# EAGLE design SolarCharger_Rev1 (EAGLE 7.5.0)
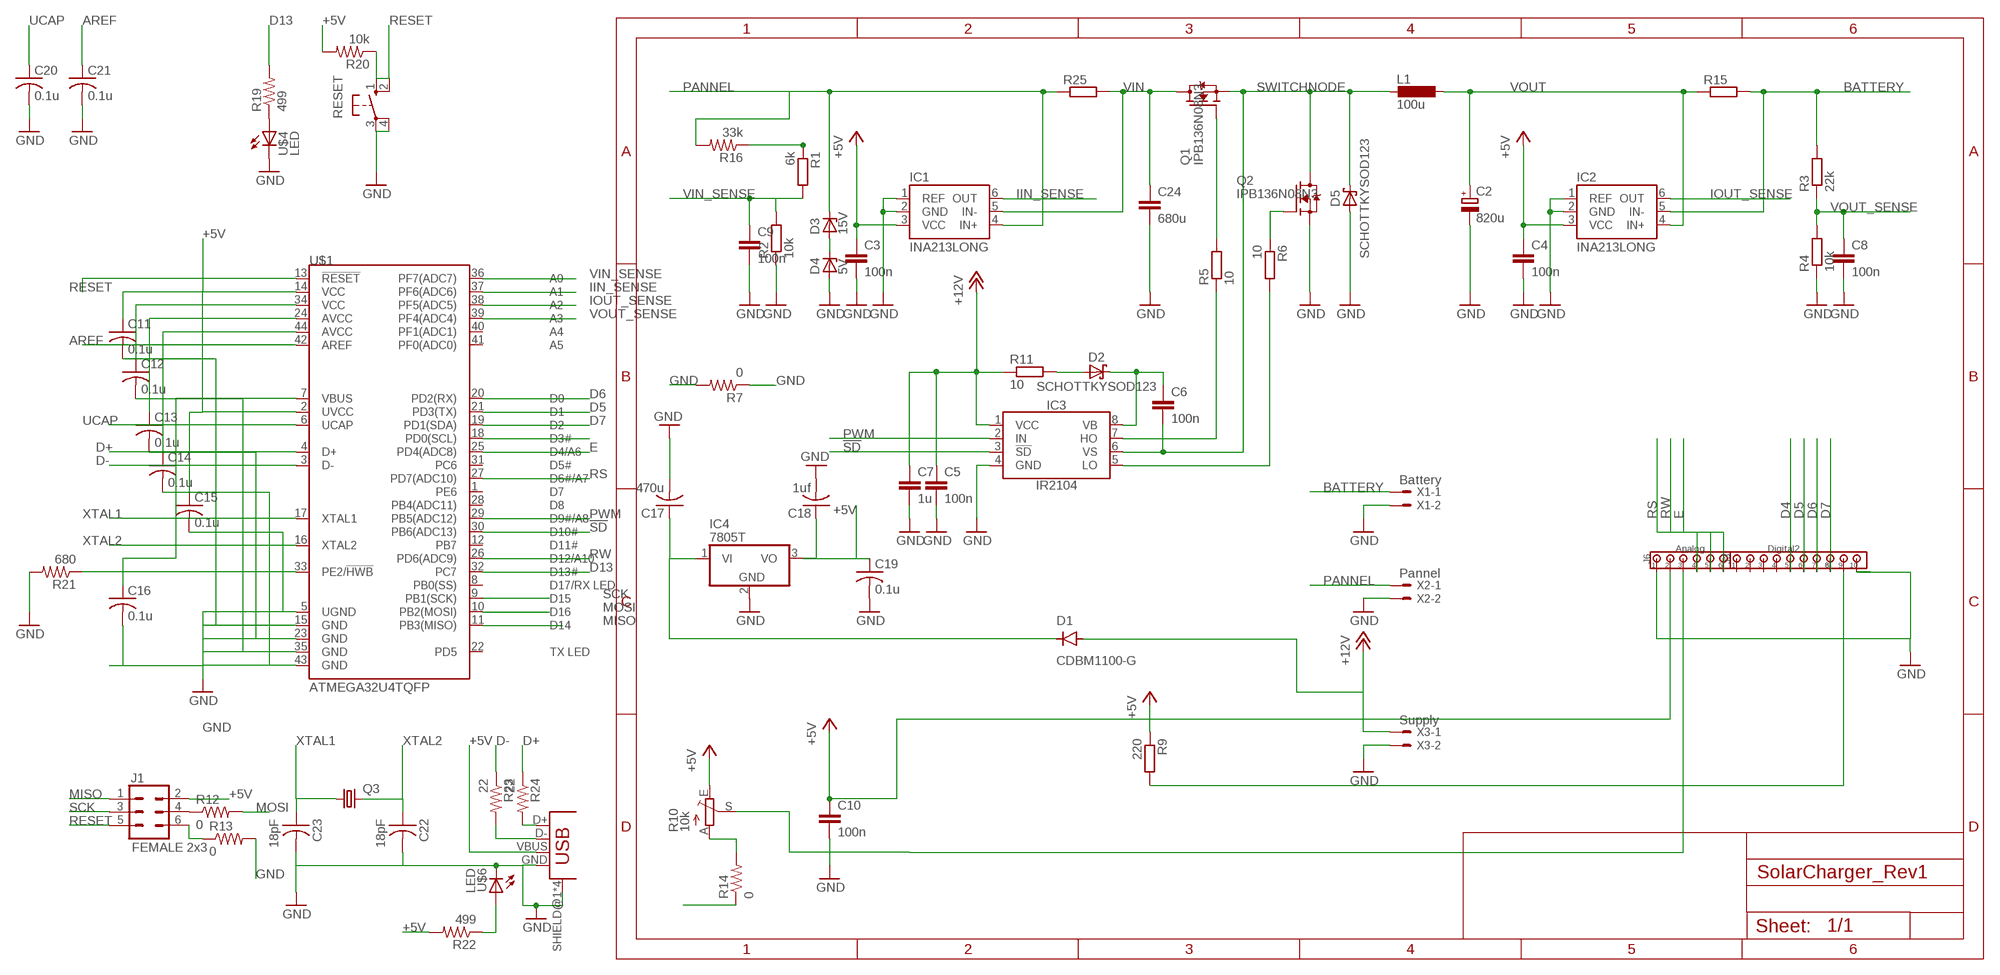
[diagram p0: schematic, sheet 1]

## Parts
C2  820u  C_POLARIZED10MM  [10MM]
C3  100n  CC0805  [C0805]
C4  100n  CC0805  [C0805]
C5  100n  CC0805  [C0805]
C6  100n  CC0805  [C0805]
C7  1u  CC0805  [C0805]
C8  100n  CC0805  [C0805]
C9  100n  CC0805  [C0805]
C10  100n  CC0805  [C0805]
C11  0.1u  C-USC1206  [C1206]
C12  0.1u  C-USC1206  [C1206]
C13  0.1u  C-USC1206  [C1206]
C14  0.1u  C-USC1206  [C1206]
C15  0.1u  C-USC1206  [C1206]
C16  0.1u  C-USC1206  [C1206]
C17  470u  C-USC1206  [C1206]
C18  1uf  C-USC1206  [C1206]
C19  0.1u  C-USC1206  [C1206]
C20  0.1u  C-USC1206  [C1206]
C21  0.1u  C-USC1206  [C1206]
C22  18pF  CAP-US1206FAB  [C1206FAB]
C23  18pF  CAP-US1206FAB  [C1206FAB]
C24  680u  10NF-PTH-10MM-10000V-1-%  [CAP-PTH-10MM]
D1  CDBM1100-G  [MINI-SMA]
D2  SCHOTTKYSOD123  [SOD123]
D3  15V  ZENER-DIODEDO41Z10  [DO41Z10]
D4  5V  ZENER-DIODEDO41Z10  [DO41Z10]
D5  SCHOTTKYSOD123  [SOD123]
IC1  INA213LONG  [SC70-6_LONG]
IC2  INA213LONG  [SC70-6_LONG]
IC3  IR2104  [SOIC8]
IC4  7805T  [TO220H]
J1  FEMALE 2x3  CONN_03X2FEMALE  [2X3]
J3  Digital2  100MIL_10X  [100MIL_10X_ROUND]
J6  Analog  100MIL_6X  [100MIL_6X_ROUND]
L1  100u  L-EU0207/12  [0207/12]
Q1  IPB136N08N3  N-PWR-MOSFETTO263-3  [TO263-3]
Q2  IPB136N08N3  IPB136N08N3_GTO263  [TO263-3@1]
Q3  CRYSTALTC26V  [TC26V]
R1  6k  R-EU_M1206  [M1206]
R2  10k  R-EU_M1206  [M1206]
R3  22k  R-EU_M1206  [M1206]
R4  10k  R-EU_M1206  [M1206]
R5  10  R-EU_M1206  [M1206]
R6  10  R-EU_M1206  [M1206]
R7  0  RES-US1206FAB  [R1206FAB]
R9  220  R-EU_M1206  [M1206]
R10  10k  TRIM_EU-B25X  [B25X]
R11  10  R-EU_M1206  [M1206]
R12  0  RES-US1206FAB  [R1206FAB]
R13  0  RES-US1206FAB  [R1206FAB]
R14  0  RES-US1206FAB  [R1206FAB]
R15  SMR  [SMR]
R16  33k  RES-US1206FAB  [R1206FAB]
R19  499  RES-US1206  [R1206]
R20  10k  RES-US1206  [R1206]
R21  680  RES-US1206  [R1206]
R22  499  RES-US1206  [R1206]
R23  22  RES-US1206  [R1206]
R24  22  RES-US1206  [R1206]
R25  SMR  [SMR]
RESET  10-XX  [B3F-10XX]
U$1  ATMEGA32U4TQFP  [SPARKFUN-DIGITALIC_TQFP44]
U$4  LED  [LED1206]
U$5  USB_MINIB  [USB_MINIB]
U$6  LED  [LED1206]
X1  Battery  22-23-2021200MIL  [200MIL_2X]
X2  Pannel  22-23-2021200MIL  [200MIL_2X]
X3  Supply  22-23-2021100MIL  [22-23-2021]

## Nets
!SD!: IC3.3(!SD!) U$1.30(PB6(ADC13))
+5V: C3.1 C4.1 C10.1 C11.1 C12.1 C13.1 C14.1 C15.1 C16.1 C18.1 C19.1 IC1.3(VCC) IC2.3(VCC) IC4.3(VO) J1.2 J6.2 R9.1 R10.E R20.2 R22.2 U$1.2(UVCC) U$1.7(VBUS) U$1.14(VCC) U$1.24(AVCC) U$1.34(VCC) U$1.44(AVCC) U$5.VBUS
+12V: C5.1 C7.1 D1.ANODE IC3.1(VCC) R11.1 X3.1
AREF: C21.1 U$1.42(AREF)
BATTERY: IC2.5(IN-) R3.2 R15.1 X1.1
D4: J3.5 U$1.18(PD0(SCL))
D5: J3.6 U$1.21(PD3(TX))
D6: J3.7 U$1.20(PD2(RX))
D7: J3.8 U$1.19(PD1(SDA))
D13: R19.2 U$1.32(PC7)
D+: R24.1 U$1.4(D+)
D-: R23.1 U$1.3(D-)
E: J6.6 U$1.25(PD4(ADC8))
GND: C2.- C3.2 C4.2 C5.2 C7.2 C8.2 C9.2 C10.2 C11.2 C12.2 C13.2 C14.2 C15.2 C16.2 C17.2 C18.2 C19.2 C20.2 C21.2 C22.2 C23.2 C24.2 D4.A D5.A IC1.1(REF) IC1.2(GND) IC2.1(REF) IC2.2(GND) IC3.4(GND) IC4.2(GND) J3.10 J6.1 Q2.3(S) R2.1 R4.1 R7.1 R7.2 R10.A R13.2 R14.1 R14.2 R21.2 RESET.3(P) RESET.4(P1) U$1.5(UGND) U$1.15(GND) U$1.23(GND) U$1.35(GND) U$1.43(GND) U$4.2(C) U$5.GND U$5.SHIELD@1(SHIELD) U$5.SHIELD@2(SHIELD) U$5.SHIELD@3(SHIELD) U$5.SHIELD@4(SHIELD) U$6.2(C) X1.2 X2.2 X3.2
IIN_SENSE: IC1.6(OUT) U$1.37(PF6(ADC6))
IOUT_SENSE: IC2.6(OUT) U$1.38(PF5(ADC5))
MISO: J1.1 U$1.11(PB3(MISO))
MOSI: R12.2 U$1.10(PB2(MOSI))
N$1: J1.4 R12.1
N$2: J1.6 R13.1
N$4: Q1.1(G) R5.2
N$7: Q2.1(G) R6.1
N$9: J3.9 R9.2
N$10: J6.3 R10.S
N$11: D2.A R11.2
N$12: C6.1 D2.C IC3.8(VB)
N$14: IC3.7(HO) R5.1
N$15: IC3.5(LO) R6.2
N$17: R1.1 R16.1
N$19: D3.A D4.C
N$20: C17.1 D1.KATHODE IC4.1(VI)
N$23: R19.1 U$4.1(A)
N$24: R21.1 U$1.33(PE2/!HWB)
N$25: R24.2 U$5.D+
N$26: R22.1 U$6.1(A)
N$27: R23.2 U$5.D-
PANNEL: D3.C IC1.4(IN+) R16.2 R25.2 X2.1
PWM: IC3.2(IN) U$1.29(PB5(ADC12))
RESET: J1.5 R20.1 RESET.1(S) RESET.2(S1) U$1.13(!RESET)
RS: J6.4 U$1.27(PD7(ADC10))
RW: J6.5 U$1.26(PD6(ADC9))
SCK: J1.3 U$1.9(PB1(SCK))
SWITCHNODE: C6.2 D5.C IC3.6(VS) L1.2 Q1.3(S) Q2.TAB(D)
UCAP: C20.1 U$1.6(UCAP)
VIN: C24.1 IC1.5(IN-) Q1.TAB(D) R25.1
VIN_SENSE: C9.1 R1.2 R2.2 U$1.36(PF7(ADC7))
VOUT: C2.+ IC2.4(IN+) L1.1 R15.2
VOUT_SENSE: C8.1 R3.1 R4.2 U$1.39(PF4(ADC4))
XTAL1: C23.1 Q3.1 U$1.17(XTAL1)
XTAL2: C22.1 Q3.2 U$1.16(XTAL2)
Unconnected: J3.1 J3.2 J3.3 J3.4 U$1.1(PE6) U$1.8(PB0(SS)) U$1.12(PB7) U$1.22(PD5) U$1.28(PB4(ADC11)) U$1.31(PC6) U$1.40(PF1(ADC1)) U$1.41(PF0(ADC0))

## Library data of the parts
C2 = 00Capacitor:C_POLARIZED
C3-C10 = 00Capacitor:C: Capacitor
C11-C21 = rcl:C-US: CAPACITOR, American symbol
C22 C23 = fab:CAP-US
C24 = SparkFun-Capacitors:10NF: 0.01uF/10nF/10,000pF ceramic capacitors; PROD_ID: CAP-09321; VALUE: 10nF
D1 = fab:CDBM1100-G: Diode schottky 100V 1A mini-SMA as found in the fablab inventory
D2 D5 = 00Diode:SCHOTTKY
D3 D4 = diode:ZENER-DIODE: Z-Diode
IC1 IC2 = 00Sensor:INA21*: Current-Shunt Monitors Voltage Output, Low- or High-Side Measurement, Bidirectional, Zero-Drift Series; GAIN: 50
IC3 = 00Logic:IR2104: Half-Bridge Driver Up to +600V Gate drive supply 10-20V Deadtime 520ns
IC4 = linear:78*: Positive VOLTAGE REGULATOR Source: http://cache.national.com/ds/LM/LM78L05.pdf http://www.fairchildsemi.com/ds/LM/LM7805.pdf
J1 = SparkFun-Connectors:CONN_03X2: Multi connection point. Often used as Generic Header-pin footprint for 0.1 inch spaced/style header connections You can populate with any combo of single row headers, but if you'd like an exact match, check these: Header - 2x3 (Male, 0.1") (PRT-12807) Header - 2x3 (Female, 0.1") (PRT-13010) 2x3 Pin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; PROD_ID: CONN-11566
J3 = 00Connector:100MIL_10X: 100mil 10-pin connector
J6 = 00Connector:100MIL_6X: 100 mil 6-pin connector
L1 = rcl:L-EU: INDUCTOR, European symbol
Q1 = 00Mosfet:N-PWR-MOSFET
Q2 = 00Mosfet:IPB136N08N3_G
Q3 = adafruit:CRYSTAL: CRYSTAL; OC_FARNELL: unknown; OC_NEWARK: unknown
R1-R6 R9 R11 = rcl:R-EU_: RESISTOR, European symbol
R7 R12-R14 R16 R19-R24 = fab:RES-US: Resistor (US Symbol)
R10 = pot:TRIM_EU-: POTENTIOMETER
R15 R25 = resistor-shunt:SMR: SMD SHUNT RESISTOR; OC_FARNELL: unknown; OC_NEWARK: unknown
RESET = switch-omron:10-XX: OMRON SWITCH; MPN: B3F-1000; OC_FARNELL: 176432; OC_NEWARK: 36M3542
U$1 = SparkFun-Retired:ATMEGA32U4: Atmel 44-pin 8-bit Microcontroller with 32KBytes of ISP Flash and USB Controller ----- Please use the QFN-44-NOPAD_1:1 package for the footprint of all boards using a 32U4. Route traces directly away from the pads as much as possible.; PROD_ID: IC-11161
U$4 U$6 = fab:LED: LED
U$5 = fab:USB_MINIB
X1 X2 = 00Connector:22-23-2021: .100" (2.54mm) Center Header - 2 Pin
X3 = 00Connector:22-23-2021: .100" (2.54mm) Center Header - 2 Pin; MF: MOLEX; MPN: 22-23-2021; OC_FARNELL: 1462926; OC_NEWARK: 25C3832

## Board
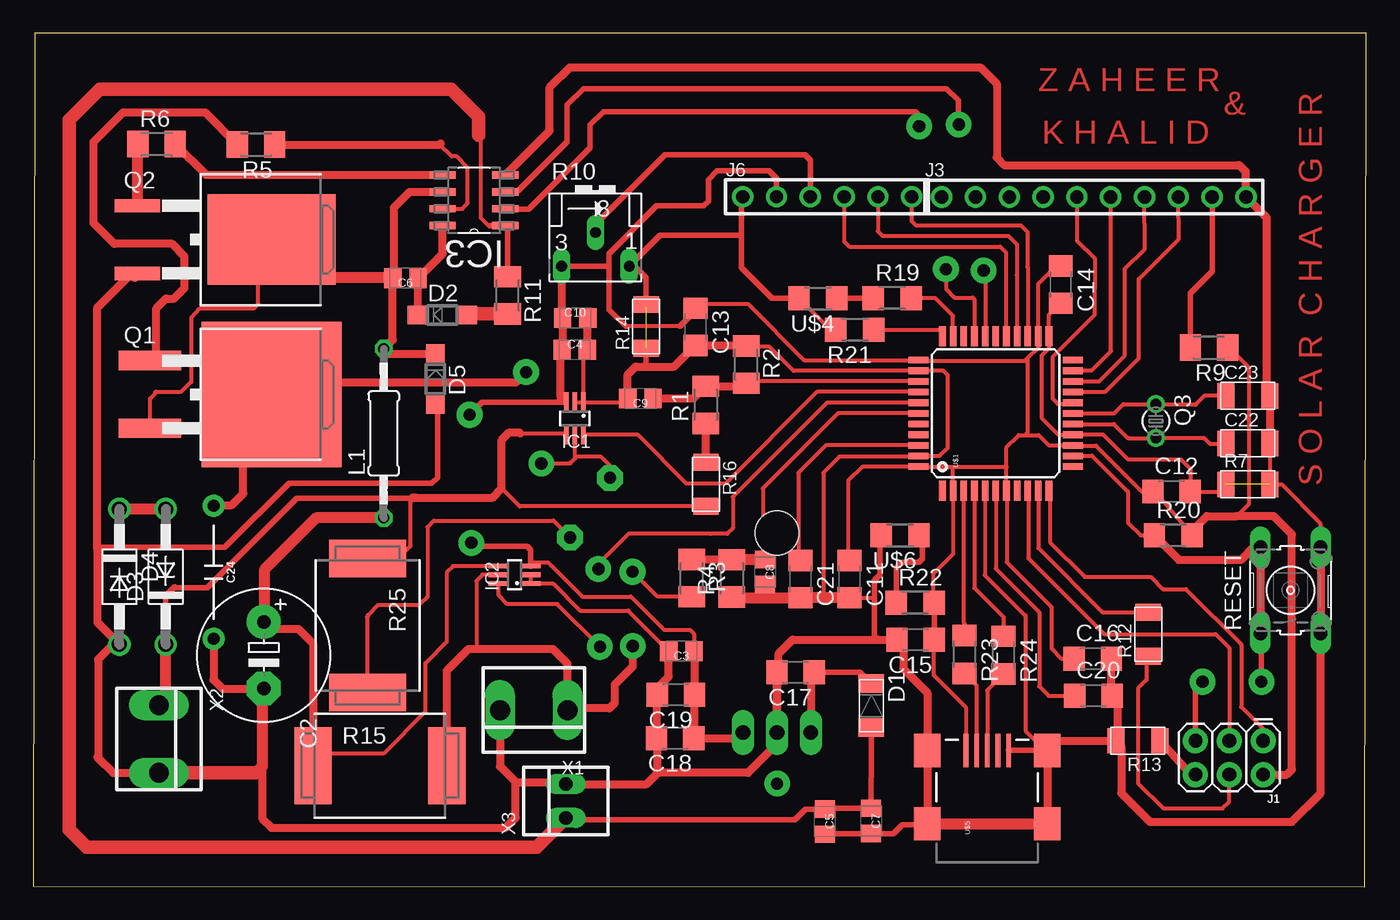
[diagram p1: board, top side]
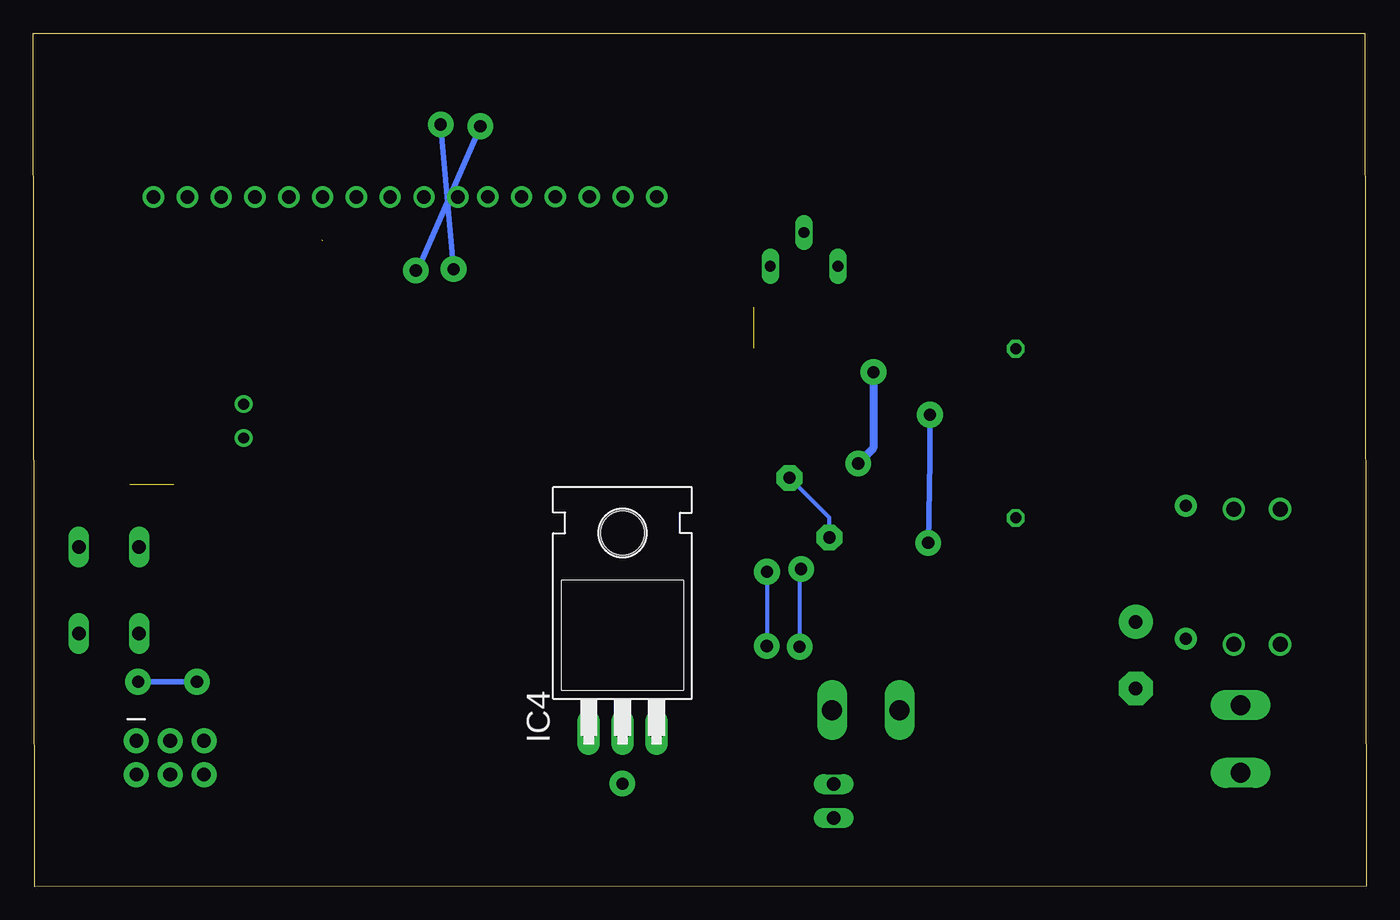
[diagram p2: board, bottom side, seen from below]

Size 100.15 x 64.08 mm. Coordinates in mm from the lower left corner, seen from the top.
Outline: 0,0.01 100.03,0 100.14,64.07 0.12,64.08 0,0.01
Copper layers (1*16): Top 0.035mm / dielectric 1.5mm / Bottom 0.035mm
Design rules "default": minimum track width 10mil, minimum drill 24mil, track to track 8mil, track to pad 8mil, pad to pad 8mil, via to via 8mil, smd to smd 8mil, copper to edge 40mil, drill to drill 8mil, minimum pad ring 10mil, minimum via ring 8mil, stop-mask expansion 4mil, vias tented up to drill 0mil, thermal gap 10mil

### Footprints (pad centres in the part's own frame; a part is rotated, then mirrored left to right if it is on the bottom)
10MM = drill 1.016 pad 2.54: + -2.5,0 | drill 1.016 pad 2.54 octagon: - 2.5,0
C0805 = smd 1.3 x 1.5: 1 -0.95,0; 2 0.95,0
C1206 = smd 1.6 x 1.8: 1 -1.4,0; 2 1.4,0
C1206FAB = smd 1.27 x 1.905: 1 -1.651,0; 2 1.651,0
CAP-PTH-10MM = drill 0.9 pad 1.651: 1 -5,0; 2 5,0
MINI-SMA = smd 1.4 x 1.9: ANODE 1.65,0; KATHODE -1.65,0
SOD123 = smd 1.4 x 1.4: A 1.9,0; C -1.9,0
DO41Z10 = drill 1.118: A 5.08,0; C -5.08,0
SC70-6_LONG = smd 0.35 x 1.5: 1 -0.65,-1.2; 2 0,-1.2; 3 0.65,-1.2; 4 0.65,1.2; 5 0,1.2; 6 -0.65,1.2
SOIC8 = smd 1.981 x 0.559: 1 -2.362,1.905; 2 -2.362,0.635; 3 -2.362,-0.635; 4 -2.362,-1.905; 5 2.362,-1.905; 6 2.362,-0.635; 7 2.362,0.635; 8 2.362,1.905
TO220H = drill 1.118 long: 1 -2.54,-10.16; 2 0,-10.16; 3 2.54,-10.16 | hole 3.302: 0,4.826
2X3 = drill 1.016 pad 1.88: 1 0,0; 2 0,2.54; 3 2.54,0; 4 2.54,2.54; 5 5.08,0; 6 5.08,2.54
100MIL_10X_ROUND = drill 1 pad 1.6: 1 -8.89,0; 2 -6.35,0; 3 -3.81,0; 4 -1.27,0; 5 1.27,0; 6 3.81,0; 7 6.35,0; 8 8.89,0; 9 11.43,0; 10 13.97,0
100MIL_6X_ROUND = drill 1 pad 1.6: 1 -6.35,0; 2 -3.81,0; 3 -1.27,0; 4 1.27,0; 5 3.81,0; 6 6.35,0
0207/12 = drill 0.813 octagon: 1 -6.35,0; 2 6.35,0
TO263-3 = smd 1.45 x 4.7: 1 -2.54,-5.65; 3 2.54,-5.65 | smd 10.9 x 10.5: TAB 0,3.5
TO263-3@1 = smd 1 x 3.4: 1 -2.54,-6.6; 3 2.54,-6.6 | smd 6.8 x 9.6: TAB 0,3.5
TC26V = drill 0.813: 1 -1.27,0; 2 1.27,0
M1206 = smd 1.6 x 2: 1 -1.4,0; 2 1.4,0
R1206FAB = smd 1.27 x 1.905: 1 -1.651,0; 2 1.651,0
B25X = drill 0.813 long: A 2.54,-1.905; E -2.54,-1.905; S 0,0.635
SMR = smd 2.8 x 5.8: 1 5.029,0; 2 -5.029,0
R1206 = smd 1.6 x 1.803: 1 -1.422,0; 2 1.422,0
B3F-10XX = drill 1.016 long: 1 -3.251,2.261; 2 3.251,2.261; 3 -3.251,-2.261; 4 3.251,-2.261
SPARKFUN-DIGITALIC_TQFP44 = smd 1.5 x 0.5: 1 -5.8,4; 2 -5.8,3.2; 3 -5.8,2.4; 4 -5.8,1.6; 5 -5.8,0.8; 6 -5.8,0; 7 -5.8,-0.8; 8 -5.8,-1.6; 9 -5.8,-2.4; 10 -5.8,-3.2; 11 -5.8,-4; 23 5.8,-4; 24 5.8,-3.2; 25 5.8,-2.4; 26 5.8,-1.6; 27 5.8,-0.8; 28 5.8,0; 29 5.8,0.8; 30 5.8,1.6; 31 5.8,2.4; 32 5.8,3.2; 33 5.8,4 | smd 0.5 x 1.5: 12 -4,-5.8; 13 -3.2,-5.8; 14 -2.4,-5.8; 15 -1.6,-5.8; 16 -0.8,-5.8; 17 0,-5.8; 18 0.8,-5.8; 19 1.6,-5.8; 20 2.4,-5.8; 21 3.2,-5.8; 22 4,-5.8; 34 4,5.8; 35 3.2,5.8; 36 2.4,5.8; 37 1.6,5.8; 38 0.8,5.8; 39 0,5.8; 40 -0.8,5.8; 41 -1.6,5.8; 42 -2.4,5.8; 43 -3.2,5.8; 44 -4,5.8
LED1206 = smd 1.6 x 1.803: 1 -1.422,0; 2 1.422,0
USB_MINIB = smd 2.5 x 0.35: D+ 3.77,0; D- 3.77,0.8; GND 3.77,-1.6; ID 3.77,-0.8; VBUS 3.77,1.6 | smd 2.5 x 2: SHIELD@1 -1.73,-4.5; SHIELD@2 -1.73,4.5; SHIELD@3 3.77,4.5; SHIELD@4 3.77,-4.5
200MIL_2X = drill 1.5 long: 1 -2.54,0; 2 2.54,0
22-23-2021 = drill 1 long: 1 -1.27,0; 2 1.27,0

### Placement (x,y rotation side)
C2  17.31,17.38 270 top
C3  48.69,17.68 180 top
C4  40.68,40.31 0 top
C5  59.47,4.88 270 top
C6  27.96,45.69 180 top
C7  62.95,4.92 270 top
C8  54.98,23.62 270 top
C9  45.61,36.65 180 top
C10  40.71,42.7 0 top
C11  61.33,23.09 270 top
C12  85.52,29.67 0 top
C13  49.75,42.04 270 top
C14  77.18,45.21 270 top
C15  66.29,18.54 180 top
C16  79.6,17.12 0 top
C17  57.27,16.1 180 top
C18  48.23,11.15 180 top
C19  48.28,14.4 180 top
C20  79.65,14.33 0 top
C21  57.63,23.09 270 top
C22  91.26,33.28 0 top
C23  91.24,36.84 0 top
C24  13.55,23.6 270 top
D1  62.96,13.59 270 top
D2  30.73,42.93 0 top
D3  9.95,23.27 90 top
D4  6.47,23.27 270 top
D5  30.22,38.13 270 top
IC1  40.68,35.15 180 top
IC2  36.16,23.42 90 top
IC3  33.11,51.54 180 top
IC4  55.87,21.72 0 bottom
J1  92.4,10.95 180 top
J3  77.14,51.79 0 top
J6  59.64,51.8 0 top
L1  26.33,34.04 90 top
Q1  14.42,36.96 270 top
Q2  14.42,48.59 270 top
Q3  84.34,34.96 270 top
R1  50.51,36.17 90 top
R2  53.56,39.19 270 top
R3  49.47,23.16 270 top
R4  52.47,23.14 90 top
R5  16.73,55.73 180 top
R6  9.26,55.75 0 top
R7  91.25,30.2 0 top
R9  88.33,40.49 180 top
R10  42.23,48.49 0 top
R11  35.63,44.4 270 top
R12  83.76,18.95 90 top
R13  83,10.95 180 top
R14  46.04,42.06 90 top
R15  26.05,9.07 0 top
R16  50.54,30.2 270 top
R19  64.53,44.2 0 top
R20  85.64,26.37 0 top
R21  61.72,41.83 180 top
R22  66.26,21.31 0 top
R23  69.97,17.42 270 top
R24  72.89,17.37 270 top
R25  25.11,19.6 270 top
RESET  94.46,22.25 90 top
U$1  72.31,35.53 90 top
U$4  58.95,44.17 180 top
U$5  71.67,6.45 90 top
U$6  65.12,26.39 180 top
X1  37.6,13.24 180 top
X2  9.44,11.07 270 top
X3  40.02,6.42 90 top

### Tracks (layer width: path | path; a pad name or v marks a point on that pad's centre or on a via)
!SD!  (via drill 0.91 pad 1.93)
  Top 0.305: v68.57,46.37 68.57,44.88 69.22,44.22 70.58,44.22 70.7,44.11 70.7,41.35 U$1.30
  Top 0.406: IC3.3 35.53,52.22 36.39,52.22 40.12,55.95 40.12,58.71 41.33,59.93 68.61,59.93 69.5,59.04 69.5,57.03 v69.53,57.23
  Bottom 0.406: v68.57,46.37 v69.53,57.23
+5V  (via drill 0.91 pad 1.93)
  Top 0.305: U$1.7 73.12,29.72 | 84.11,29.7 C12.1 | U$5.VBUS 70.1,10.25 70.1,13.44 67.66,15.88 67.66,18.47 67.25,18.88 C15.1 | C14.1 76.86,46.61 75.51,45.26 U$1.24 75.53,41.31 75.53,40.51 74.7,39.68 | 73.12,29.72 73.14,29.7 73.14,24.36 76.5,21.01 76.5,17.88 77.26,17.12 C16.1 | 73.12,29.72 73.12,31.52 | 73.12,31.52 73.12,32.99 74.03,33.91 74.51,33.91 | 74.51,33.91 75.53,33.91 76.31,33.13 U$1.14 78.12,33.12 79.85,33.12 83.31,29.67 C12.1 | 66.52,31.53 66.52,31.52 69.08,31.52 | 69.08,31.52 73.12,31.52 | 69.08,31.52 69.08,29.76 U$1.2 69.11,24.96 67.6,23.46 67.6,21.39 R22.2 | 90.42,27.81 91.31,28.7 91.31,35.05 91.31,35.14 91.31,39 89.83,40.49 R9.1 | C11.1 61.33,25.15 61.23,25.26 61.23,30.47 62.28,31.53 66.52,31.53 | 66.52,31.53 U$1.44 | C13.1 50.33,43.76 53.69,43.76 57.92,39.53 U$1.34 66.57,39.47 74.49,39.47 74.7,39.68 | 39.73,36.65 IC1.3 | 49.55,17.76 C3.1 49.63,18.99 49.34,19.28 47.39,19.28 44.9,21.77 41.25,21.77 38.95,24.07 38.95,24.09 38.93,24.09 38.69,24.33 37.63,24.33 IC2.3 | 39.59,36.86 39.47,36.73 39.47,36.35 | 37.7,24.07 IC2.3 | 34.9,25.57 34.92,25.55 | C12.1 84.44,29.67 84.44,29.46 R20.2 | IC2.3 | 37.38,24.99 37.37,25 | 48.59,42.06 44.52,42.06 | 74.7,39.68 74.7,34.1 74.51,33.91
  Top 0.406: R22.2 C15.1 | v32.78,35.43 33.7,36.35 39.47,36.35 IC1.3 | 43.25,46.63 43.25,47.52 46.84,51.11 50.36,51.11 50.71,51.47 50.71,53.09 51.36,53.74 55.29,53.74 55.83,53.19 J6.2 | 44.52,42.06 43.25,43.33 43.25,46.63 | R10.E 43.2,46.58 43.25,46.63 | C13.1 49.75,43.23 48.59,42.06 | 34.9,25.57 33.21,25.57 33.1,25.68 v32.91,25.81 | 34.92,25.55 37.1,25.55 37.37,25.29 37.37,25 IC2.3
  Top 0.61: R10.E 39.69,42.76 C10.1 39.76,40.34 C4.1 39.59,40.17 39.59,36.86 | R20.2 87.06,26.72 88.16,27.81 90.42,27.81 93.19,27.81 94.56,26.44 94.56,8.79 94.18,8.41 J1.2 | IC4.3 52.92,11.15 C18.1 49.63,14.35 C19.1 49.68,17.68 C3.1
  Bottom 0.406: v32.91,25.81 32.78,32 v32.78,35.43
+12V
  Top 0.305: 34.28,49.63 34.38,49.63 34.42,49.59 34.23,49.59 33.63,50.2 33.63,56.28 33.55,56.36
  Top 0.406: D1.ANODE 62.96,10.4 C7.1 59.47,5.87 C5.1 59.45,5.81 58.03,5.81 57.23,5.01 40.16,5.01 | 33.47,56.44 33.55,56.36 | 34.28,49.63 IC3.1 35.63,49.48 R11.1
  Top 0.61: X3.1
  Top 1.016: 33.47,56.44 33.47,57.81 31.39,59.89 5,59.89 2.69,57.58 2.69,4.27 4.01,2.95 37.82,2.95 X3.1 | 39.85,4.98 X3.1 | 40.16,5.01 X3.1
AREF
  Top 0.305: 57.65,24.51 C21.1 57.48,24.63 57.48,31.07 59.55,33.13 U$1.42
BATTERY  (via drill 0.9, 0.91 pad 1.93)
  Top 0.305: R3.2 46.91,21.76 v45.03,23.65 | IC2.5 33.75,23.42 33.29,22.96 33.29,18.04 33.1,17.85
  Top 0.61: v45.04,18.07 45.04,16.52 43.68,15.17 43.68,13.78 43.29,13.38 40.27,13.38 X1.1 40.13,16.74 39.03,17.85 33.1,17.85 32.69,17.85 31.08,16.23 R15.1
  Bottom 0.305: v45.03,18.06 v45.03,23.65 v45.04,23.64 v45.04,18.07
D4  (1 unrouted)
  Top 0.305: 78.43,48.59 78.43,48.58 | J3.5 78.42,48.5 79.75,47.17 79.75,44.84 | U$1.18 78.02,36.25 76.97,36.25 76.57,36.65 76.57,39.74 79.75,42.92 79.75,44.84 | 79.75,44.84 79.77,45.03
D5
  Top 0.305: U$1.21 78.13,38.76 79.52,38.76 80.97,40.21 J3.6
D6
  Top 0.305: U$1.20 80.08,37.95 82.01,39.88 82.01,46.38 83.51,47.88 J3.7
D7
  Top 0.305: U$1.19 78.13,37.16 80.54,37.16 83.05,39.67 83.05,45.62 86.05,48.62 J3.8
D13
  Top 0.305: U$1.32 69.11,42.85 67.76,44.2 R19.2
D+
  Top 0.305: U$1.4 | U$1.4 70.71,22.43 72.89,20.24 R24.1
D-
  Top 0.305: U$1.3 69.89,29.72 69.89,19.81 69.97,19.74 R23.1
E
  Top 0.305: U$1.25 74.71,46.5 74.67,46.53 74.67,49.19 74.22,49.65 66.33,49.65 65.99,49.99 J6.6
GND  (2 unrouted)
  Top 0.305: U$1.43 | U$1.43 67.03,32.33 | 67.03,32.33 68.09,32.33 68.7,32.94 68.7,38.4 68.37,38.73 U$1.35 57.12,38.73 55.31,40.54 53.62,40.54 R2.1 | C12.2 | U$1.5 71.49,29.72 71.49,23.39 74.54,20.35 74.54,11.71 76.03,10.22 U$5.SHIELD@4 | C11.2 63.19,21.69 63.21,21.72 | C21.2 58.89,21.69 | 66.46,32.28 U$1.43 | R21.2 59.78,41.91 U$4.2 | IC1.2 IC1.1 | IC1.1 44.36,36.35 C9.2 | IC1.1 41.33,40.01 C4.2 | C3.2 44.69,20.73 41.09,20.73 39.05,22.77 IC2.1 IC2.2 | C14.2 76.31,42.94 U$1.23 76.32,41.32 76.32,40.43 75.76,39.87 75.76,35.21 77.03,33.93 U$1.15 80.38,33.93 82.24,32.08 86.22,32.08 86.94,31.36 86.94,29.69 C12.2 | 59.52,21.69 59.35,21.85 59.35,31.07 60.56,32.28 66.98,32.28 67.03,32.33 | C12.2 89.06,29.67 R7.1 | 92.89,32.9 R7.2 93.79,30.2 96.69,27.3 96.69,25.53 RESET.4
  Top 0.406: U$5.GND U$5.SHIELD@4 | C22.2 92.53,33.02 | U$5.SHIELD@3 67.15,10.2 67.15,4.62 65.29,4.62 64.62,3.95 62.97,3.95 C7.2 59.08,3.97 58.92,3.82 59.35,3.82 C5.2 | C10.2 41.66,40.47 41.6,40.41 | R14.1 46.04,39.17 45.92,39.04 | U$4.2 55.5,44.18 53.2,46.48 53.2,48.87 | D5.A 30.32,36.23 30.63,35.92 30.61,35.92 30.36,35.67 30.36,30.71 29.94,30.29 19.21,30.29 14.4,25.48 4.95,25.48 4.82,25.35 | R14.2 46.04,43.49 46.04,45.71 45.16,46.58 R10.A 47.09,48.9 53.17,48.9 53.2,48.87 | 59.78,41.91 59.78,42.31 | 63.21,26.41 U$6.2 63.62,26.31 63.62,23.4 63.21,22.99 63.21,21.72 63.21,18.78 63.45,18.54 | 53.2,48.87 53.2,51.7 J6.1 | J3.10 91.07,51.83
  Top 0.61: U$5.SHIELD@4 U$5.SHIELD@1 | U$5.SHIELD@2 U$5.SHIELD@3 67.17,14.56 65.37,16.36 65.37,18.06 C15.2 63.45,18.54 57.04,18.54 56,17.5 56,16.54 55.92,16.46 55.92,11.64 55.87,11.59 | 55.87,11.59 C17.2 | 46.83,11.68 46.83,14.35 C19.2 46.63,14.65 47.73,15.76 C3.2 47.48,17.42 | 46.83,11.68 C18.2 46.88,11.1 | U$5.SHIELD@4 76.4,10.45 76.4,10.44 76.91,10.95 R13.2 | C8.2 54.98,22.2 55.52,21.67 57.6,21.67 C21.2 | C4.2 41.63,42.67 C10.2 | C9.2 44.66,38.45 45.26,39.04 45.92,39.04 48.16,39.04 C13.2 53.52,40.64 R2.1 | 46.83,11.68 46.88,11.63 46.88,8.64 46.83,8.59 46.85,8.56 46.95,8.56 | 7.64,45.69 7.64,45.87 Q2.3 7.38,46.05 4.82,43.48 4.82,25.35 4.82,19.84 D4.A 6,18.19 4.88,17.06 4.88,9.77 4.82,9.71 6,8.54 X2.2 | 81.07,17.2 C16.2 81,14.38 C20.2 81.05,14.17 81.48,13.74 81.48,11.05 R13.2 | RESET.4 RESET.3 96.72,7.01 94.56,4.85 83.89,4.85 81.73,7.01 81.73,10.54 81.45,10.82 R13.2 | 76.14,10.82 76.17,10.79 U$5.SHIELD@4 | 92.53,33.02 92.64,33.14 | 55.87,11.59 IC4.2 | IC4.2 | X3.2 40.61,7.69 | 40.61,7.69 46.08,7.69 46.95,8.56 | X1.2 35.05,9.03 36.26,7.83 | 36.26,7.83 40.48,7.83 40.61,7.69 | 17.2,9.03 17.2,5.11 17.9,4.4 35.47,4.4 36.23,5.17 36.23,7.81 36.26,7.83 | C24.2 13.55,15.52 14.21,14.86 17.3,14.86 C2.- | IC4.2 55.87,10.72 53.7,8.54 46.97,8.54 46.95,8.56 | C22.2 92.89,32.9 C23.2 92.64,37.09 92.64,50.26 J3.10 | IC3.4 38.8,56.77 38.8,60.01 40.32,61.53 71.14,61.53 72.39,60.28 72.39,54.74 72.94,54.19 90.61,54.19 91.07,53.72 91.07,51.83
  Top 0.813: 67.15,4.62 67.25,4.72 U$5.SHIELD@1 | C11.2 59.52,21.69 C21.2 52.52,21.69 R4.1 | C2.- 17.27,14.88 17.2,14.81 17.2,9.03 16.7,8.53
  Top 1.016: X2.2 16.7,8.53
IIN_SENSE
  Top 0.305: IC1.6 45.39,33.95 49.09,30.25 49.1,30.26 51.99,30.26 58.88,37.15 66.47,37.15 U$1.37
IOUT_SENSE  (via drill 0.91 pad 1.93)
  Top 0.305: U$1.38 66.49,36.35 59.64,36.35 52.57,29.27 52.57,26.92 52.13,26.49 50.87,26.49 50.86,26.48 44.71,26.48 44.7,26.48 42.46,24.24 v42.46,23.85 | v42.57,18 39.35,21.22 35.61,21.22 34.96,21.87 IC2.6
  Bottom 0.305: v42.46,23.85 42.57,23.74 v42.57,18
MISO
  Top 0.305: J1.1 92.4,11.84 90.75,13.49 90.75,18.19 86.6,22.34 84.88,22.34 83.96,23.26 79,23.26 76.4,25.86 76.4,29.65 U$1.11
MOSI
  Top 0.305: U$1.10 | 83.72,20.56 R12.2 80.34,20.6 75.51,25.43 U$1.10
N$1
  Top 0.305: R12.1 83.64,17.4 83.64,15.52 83,14.88 83,7.77 84.91,5.87 89.35,5.87 89.86,6.38 J1.4
N$2
  Top 0.61: R13.1 86.96,8.41 J1.6
N$3  (via drill 0.91 pad 1.93)
  other vias: 55.88,7.73
N$4
  Top 0.305: 9.24,39.75 9.02,39.75 Q1.1
  Top 0.61: R5.2 12.94,58.12 6.72,58.12 4.51,55.91 4.51,49.83 6.09,48.26 10.43,48.26 11.37,47.31 11.37,44.95 10.56,44.15 9.96,44.15 9.24,43.42 9.24,39.75
N$7
  Top 0.813: Q2.1 7.86,51.17 R6.1
N$9
  Top 0.406: J3.9 88.57,46.19 86.94,44.56 R9.2
N$10
  Top 0.406: J6.3 58.37,53.11 58.38,53.12 58.38,54.55 57.96,54.97 47.45,54.97 42.23,49.75 R10.S
N$11
  Top 1.016: D2.A 32.7,43 R11.2
N$12
  Top 0.61: D2.C 28.91,43.01 C6.1 30.75,47.54 IC3.8
N$14
  Top 0.305: IC3.7 32.23,50.9 32.65,51.32 32.65,53.99 31.81,54.83 31.44,54.83 30.54,55.73
  Top 0.61: 18.19,55.67 R5.1 30.54,55.73 30.62,55.8
N$15
  Top 0.61: R6.2 12.98,53.44 IC3.5
N$17
  Top 0.61: R1.1 50.51,31.63 R16.1
N$19
  Top 0.813: D3.A D4.C
N$20
  Top 0.406: D1.KATHODE 62.09,16.1 C17.1 | 58.49,15.92 58.41,15.92
  Top 0.61: C17.1 58.49,15.92 | 58.41,15.92 IC4.1
N$23
  Top 0.406: U$4.1 60.39,44.2 R19.1
N$24
  Top 0.305: 68.37,41.91 68.39,41.94 68.39,41.42 U$1.33 68.31,41.83 R21.1
N$25
  Top 0.305: R24.2 71.67,14.73 U$5.D+
N$26
  Top 0.406: R22.1 64.84,23.95 65.25,24.35 66.54,24.35 66.82,24.64 66.82,27.06 U$6.1
N$27
  Top 0.305: R23.2 70.87,15.1 U$5.D-
PANNEL
  Top 0.305: 39.94,33.86 IC1.4 39.96,34.03 36.58,34.03 | 28.35,29.05 28.35,28.91 28.31,28.87 28.31,25.55 27.53,24.76 26.16,24.76 25.62,24.23 | R16.2 36.55,28.55 35.2,29.9
  Top 0.406: 28.8,29.11 28.7,29.21 | R25.2 25.62,24.23 26.29,23.7 | 28.35,29.05 28.52,29.21 28.73,29.21 28.77,29.17 21.59,29.17 | 21.53,29.17 21.75,29.16 21.58,29.16 | D3.C 9.96,21.84 10.63,22.51 10.7,22.45 13.05,22.45 19.78,29.17 21.59,29.17 | 21.18,29.16 21.58,29.16 | 21.58,29.16 21.59,29.17
  Top 0.61: 28.52,29.21 28.7,29.21 34.51,29.21 35.2,29.9 35.2,33.55 35.75,34.1 36.51,34.1 36.58,34.03
  Top 0.813: X2.1 9.95,14.12 D3.C
PWM  (via drill 0.91 pad 1.93)
  Top 0.305: v71.4,46.27 71.4,45.8 71.53,45.67 71.53,41.36 U$1.29
  Top 0.406: IC3.2 35.53,50.85 37.21,50.85 41.85,55.49 41.85,57.22 42.83,58.2 66.27,58.2 66.69,57.78 66.69,57.24 v66.55,57.1
  Bottom 0.406: v66.55,57.1 71.53,45.67 v71.4,46.27
RESET  (via drill 0.91 pad 1.93)
  Top 0.305: U$1.13 | U$1.13 78.13,32.36 79.55,32.36 82.24,29.67 82.24,27.33 83.2,26.37 R20.1
  Top 0.406: RESET.1 92.27,18.92 v92.27,15.38 | v87.86,15.38 87.32,15.01 J1.5
  Top 0.61: R20.1 86.05,24.54 90.75,24.54 91.71,25.5 RESET.2 RESET.1
  Bottom 0.406: v92.27,15.38 v87.86,15.38
RS
  Top 0.305: U$1.27 73.11,45.22 73.08,45.24 73.08,47.63 72.65,48.06 61.3,48.06 60.91,48.45 J6.4
RW
  Top 0.305: U$1.26 73.91,45.93 73.89,45.94 73.89,48.25 73.27,48.87 63.81,48.87 63.45,49.23 J6.5
SCK
  Top 0.305: U$1.9 74.75,29.7 74.75,24.66 80.46,18.95 88.84,18.95 89.86,17.93 J1.3 89.86,11.2
SWITCHNODE
  Top 0.305: Q1.3 8.77,36.64 9.15,37.02 9.15,37.12 9.2,37.16 11.12,37.16 11.82,37.86 | 11.82,37.86 | 11.82,37.86 11.89,37.88 11.89,42.74 12.52,43.43 16.58,43.43 16.91,43.75 16.91,46.04 16.35,46.6
  Top 0.61: IC3.6 28.26,52.17 27.09,51 27.09,45.78 C6.2 27.01,41.06 L1.2 26.69,40.03 D5.C | 15.13,45.85 15.59,45.85 16.35,46.6 16.63,46.89 16.63,48.06 17.11,48.54 18.43,48.54 18.38,48.59 Q2.TAB
  Top 0.813: C6.2 26.98,45.72 17.9,45.72 17.92,45.74 Q2.TAB
UCAP
  Top 0.305: U$1.6 72.33,29.71 72.31,29.68 72.31,23.88 75.58,20.6 75.58,15.04 76.3,14.33 C20.1
VIN  (via drill 0.91 pad 1.93)
  Top 0.305: v38.17,31.78 40.3,31.78 | 40.71,32.16 40.33,31.78 40.3,31.78 | 40.71,32.16 40.71,33.93 IC1.5 | 40.3,31.78 40.27,31.81 | v43.33,30.69 43.33,31.61 42.65,32.28 40.84,32.28 40.71,32.16 | v40.34,26.21 39.07,27.47 30.09,27.47 29.62,27 29.62,21.78 28.96,21.12 25.88,21.12 25.14,20.38 25.14,20.3 25.07,20.22 25.07,14.62 R25.1
  Top 0.61: 18.08,35.69 18.48,36.09 18.56,36.17 | 18.56,36.17 20.26,37.87 36.26,37.87 v37.03,38.63 | 38.14,31.81 v38.17,31.78 | 13.74,28.64 14.91,28.64 15.78,29.5 15.78,31.98 15.79,32 16.92,32 16.98,32.06 18.09,32.06 18.1,32.06 | 18.56,36.45 18.56,36.17
  Top 1.016: 18.1,32.06 18.08,37.52 18.56,37.03 18.56,36.45 18.05,36.96 Q1.TAB | 13.65,28.56 13.66,28.56 13.69,28.59 | 13.69,28.59 13.74,28.64 | C24.1 13.67,28.6 13.69,28.59
  Bottom 0.305: v40.34,26.21 40.34,27.7 v43.33,30.69
  Bottom 0.61: v37.03,38.63 37.03,32.92 v38.17,31.78
VIN_SENSE
  Top 0.305: U$1.36 53.7,37.93 R2.2
  Top 0.61: C9.1 49.6,36.65 R1.2 53.34,37.57 R2.2
VOUT
  Top 0.305: 21.36,8.69 21.01,8.34 | IC2.4 31.54,24.07 31.06,23.6 31.06,18.37 29.48,16.78 29.45,16.78 29.45,13.12 26.32,9.99 21.28,9.99 21.01,9.71 | 21.17,8.67 21.01,8.83
  Top 0.406: 21.26,8.41 R15.2 | 21.41,8.74 21.36,8.69
  Top 0.61: 26.4,27.78 L1.1 | 17.2,19.35 19.91,19.35 21.01,18.25 21.01,10.12 21.01,9.71 21.01,8.83 21.01,8.34 R15.2
  Top 0.813: 17.37,19.78 17.53,19.68 17.2,19.35 | 17.29,19.9 C2.+ 17.36,19.92 17.36,23.77 21.27,27.69 L1.1
  Top 1.016: 17.52,20.09 C2.+ 17.34,19.94 17.37,19.78
VOUT_SENSE
  Top 0.305: 55.29,24.88 C8.1 54.81,24.75 54.81,29.9 60.45,35.53 U$1.39
  Top 0.61: R4.2 49.5,24.54 R3.1
  Top 0.813: R4.2 52.5,24.57 C8.1
XTAL1
  Top 0.305: 78.13,35.51 U$1.17 81.21,35.53 81.91,36.23 Q3.1 | Q3.1 | C23.1 87.98,36.84 87.31,36.18 84.39,36.18 Q3.1
XTAL2
  Top 0.305: 78.14,34.7 U$1.16 81.19,34.73 82.25,33.67 84.32,33.67 Q3.2 84.35,33.67 87.98,33.67 88.4,33.25 89.57,33.25 C22.1

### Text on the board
Top: Z A H E E R | & | K H A L I D | S O L A R C H A R G E R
